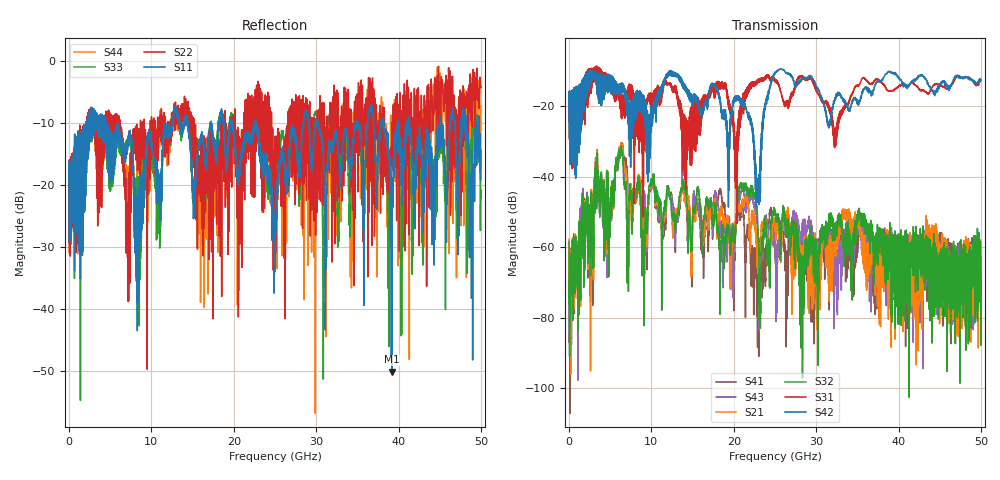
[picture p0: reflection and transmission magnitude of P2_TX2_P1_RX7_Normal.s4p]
!Keysight Technologies,N5225B,MY57041031,A.13.20.10
!Date: Friday, May 31, 2019 11:24:54
!Correction: S11(Full 4 Port(1,2,3,4))
!S12(Full 4 Port(1,2,3,4))
!S13(Full 4 Port(1,2,3,4))
!S14(Full 4 Port(1,2,3,4))
!S21(Full 4 Port(1,2,3,4))
!S22(Full 4 Port(1,2,3,4))
!S23(Full 4 Port(1,2,3,4))
!S24(Full 4 Port(1,2,3,4))
!S31(Full 4 Port(1,2,3,4))
!S32(Full 4 Port(1,2,3,4))
!S33(Full 4 Port(1,2,3,4))
!S34(Full 4 Port(1,2,3,4))
!S41(Full 4 Port(1,2,3,4))
!S42(Full 4 Port(1,2,3,4))
!S43(Full 4 Port(1,2,3,4))
!S44(Full 4 Port(1,2,3,4))
!S4P File: Measurements: <S11,S12,S13,S14>,
!<S21,S22,S23,S24>,
!<S31,S32,S33,S34>,
!<S41,S42,S43,S44>:
# Hz S  dB  R 50.0
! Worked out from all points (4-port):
!   5000 points, 10 MHz to 50 GHz, reference 50 ohm
!   strongest paths, dB at 10 MHz, 12.51 GHz, 25.01 GHz, 37.51 GHz, 50 GHz:
!     S42: -19.7, -10.0, -10.7, -12.6, -12.4
!     S31: -19.4, -14.9, -13.0, -12.4, -12.6
!     S32: -58.5, -51.2, -49.8, -65.1, -67.9
!     S21: -57.7, -52.4, -53.1, -65.7, -65.4
!     S43: -58.2, -48.0, -58.4, -59.8, -83.5
!     S41: -87.0, -46.7, -60.0, -59.7, -64.5
!   lowest |S11| = -50.1 dB at 39.22 GHz (marker M1), VSWR 1.01, Z = 49.7 + j0.0909 ohm
!   |S11| at or under -10 dB: 4.481 GHz to 11.72 GHz (7.238 GHz wide, 89.4 % of centre); 22.73 GHz to 28.43 GHz (5.704 GHz wide, 22.3 % of centre); 30.26 GHz to 34.82 GHz (4.559 GHz wide, 14 % of centre)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
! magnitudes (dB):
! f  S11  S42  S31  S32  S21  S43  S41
! 10 MHz  -19.2  -19.7  -19.4  -58.5  -57.7  -58.2  -87.0
! 6.35 GHz  -14.0  -16.6  -23.3  -31.7  -30.5  -31.5  -30.6
! 8.97 GHz  -22.7  -16.9  -25.2  -60.1  -59.9  -57.5  -52.8
! 22.93 GHz  -11.8  -40.6  -13.1  -53.9  -64.4  -58.5  -72.6
! 25.27 GHz  -20.3  -9.8  -13.0  -51.3  -54.4  -62.5  -61.2
! 39.22 GHz  -50.1  -10.6  -15.7  -62.7  -66.7  -58.1  -57.9
! 50 GHz  -14.4  -12.4  -12.6  -67.9  -65.4  -83.5  -64.5
